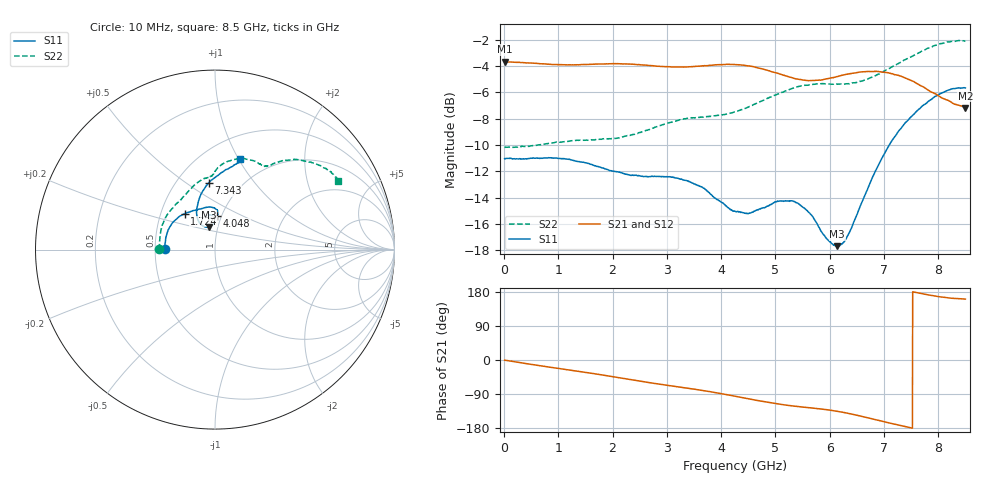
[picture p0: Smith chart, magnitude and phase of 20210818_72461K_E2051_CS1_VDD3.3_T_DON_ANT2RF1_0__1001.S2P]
!Agilent Technologies,E5071C,MY46417908,A.11.23
!Date: Wed Aug 18 14:24:02 2021
!Data & Calibration Information:
!Freq	S11:SOLT2(ON)	S21:SOLT2(ON)	S12:SOLT2(ON)	S22:SOLT2(ON)
!PortZ  Port1:50+j0  Port2:50+j0
!Above PortZ is port z conversion or system Z0 setting when saving the data.
!When reading, reference impedance value at option line is always used.
# Hz S dB R 50
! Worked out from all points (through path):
!   1601 points, 10 MHz to 8.5 GHz, reference 50 ohm
!   highest |S21| = -3.67 dB at 10 MHz (marker M1); lowest = -7.2 dB at 8.5 GHz (marker M2)
!   group delay of S21, straight-line fit = 65.8 ps
!   lowest |S11| = -17.7 dB at 6.139 GHz (marker M3), VSWR 1.30, Z = 45.2 + j11.6 ohm
!   |S11| at or under -10 dB: start of sweep to 7.097 GHz
!   |S22| runs from -10.2 to -2.1 dB; largest |S21 - S12| = 0.0033
!   S11 on the Smith chart (normalised r, x): 10 MHz: 0.56, +0.00; 1.724 GHz: 0.66, +0.28; 4.048 GHz: 0.95, +0.37; 7.343 GHz: 0.71, +0.61; 8.5 GHz: 0.73, +1.01
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1e7  -11.03 179.6  -3.67 -0.4  -3.67 -0.4  -10.14 179.9
8.37775e8  -10.97 157.7  -3.88 -18.9  -3.88 -18.9  -9.88 158.6
1.426769e9  -11.29 139.3  -3.90 -31.1  -3.90 -31.1  -9.63 141.9
1.723919e9  -11.62 130.3  -3.86 -37.6  -3.86 -37.6  -9.58 133.7
2.334138e9  -12.31 114.4  -3.87 -51.8  -3.88 -51.8  -9.26 119.9
2.843538e9  -12.39 102.5  -4.03 -63.3  -4.02 -63.3  -8.56 109.1
3.416612e9  -12.78 90.1  -4.07 -75.1  -4.06 -75.1  -7.94 98.9
4.048056e9  -14.46 86.7  -3.90 -89.9  -3.89 -90.0  -7.69 92.4
4.255e9  -15.03 89.5  -3.90 -95.6  -3.89 -95.5  -7.48 91.0
4.801544e9  -14.76 100.8  -4.28 -110.2  -4.28 -110.2  -6.57 86.3
5.289719e9  -14.23 96.8  -4.88 -120.7  -4.89 -120.7  -5.74 77.2
5.671769e9  -15.36 91.2  -5.11 -126.6  -5.12 -126.7  -5.41 69.1
5.921162e9  -16.98 93.4  -5.00 -130.6  -5.02 -130.8  -5.37 64.5
6.138719e9  -17.67 105.4  -4.82 -135.3  -4.82 -135.5  -5.39 61.6
6.297906e9  -17.13 113.9  -4.64 -139.5  -4.63 -139.7  -5.36 59.6
6.526075e9  -15.01 120.1  -4.50 -146.5  -4.48 -146.6  -5.21 58.1
6.786081e9  -12.47 115.5  -4.43 -155.3  -4.41 -155.4  -4.83 56.2
7.088538e9  -10.06 104.8  -4.54 -165.9  -4.54 -165.8  -4.21 53.2
7.343238e9  -8.58 95.5  -4.83 -174.3  -4.83 -174.3  -3.63 49.5
7.709369e9  -7.03 82.9  -5.56 174.7  -5.56 174.6  -2.84 42.6
8.054275e9  -6.08 75.5  -6.41 166.2  -6.36 166.2  -2.31 35.9
8.5e9  -5.67 74.8  -7.19 160.7  -7.14 160.9  -2.14 29.1
